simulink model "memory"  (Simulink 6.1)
settings: Solver=ode45  StartTime=0.0  StopTime=25.0  RelTol=1e-3
undefined symbols (not defined in the file or in its folder): Bit, Location, Lower, memory_netlist, Width
libraries: xbsIndex_r3 x19, adlibrary2 x2

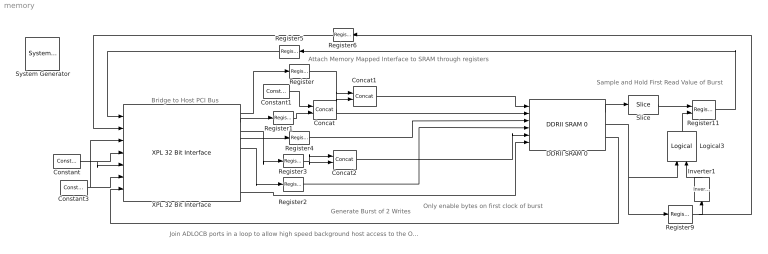
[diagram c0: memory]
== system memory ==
  note: Bridge to Host PCI Bus
  note: Attach Memory Mapped Interface to SRAM through registers
  note: Join ADLOCB ports in a loop to allow high speed background host access to the Off Chip Ram
  note: Generate Burst of 2 Writes
  note: Only enable bytes on first clock of burst
  note: Sample and Hold First Read Value of Burst
  " System Generator" : xbsIndex_r3/ System Generator  Tag=genX  xilinxfamily=Virtex2P  part=xc2vp70  speed=-6  package=ff1704  synthesis_tool=XST  directory=./memory_netlist  testbench=off  simulink_period=1  sysclk_period=10  incr_netlist=off  trim_vbits=Everywhere in SubSystem  dbl_ovrd=According to Block Masks  core_generation=According to Block Masks  run_coregen=off  deprecated_control=off  eval_field=0
  Concat : xbsIndex_r3/Concat  num_inputs=2  explicit_period=off  period=1  dbl_ovrd=off
  Concat1 : xbsIndex_r3/Concat  num_inputs=2  explicit_period=off  period=1  dbl_ovrd=off
  Concat2 : xbsIndex_r3/Concat  num_inputs=2  explicit_period=off  period=1  dbl_ovrd=off
  Constant : xbsIndex_r3/Constant  const=0  equ=P=C  arith_type=Boolean  n_bits=1  bin_pt=0  opselect=C  inp2=PCIN>>17  opr=+  inp1=P  carry=CIN  iostate=0  explicit_period=on  period=1  dbl_ovrd=off
  Constant1 : xbsIndex_r3/Constant  const=0  equ=P=C  arith_type=Unsigned  n_bits=5  bin_pt=0  opselect=C  inp2=PCIN>>17  opr=+  inp1=P  carry=CIN  iostate=0  explicit_period=on  period=1  dbl_ovrd=off
  Constant3 : xbsIndex_r3/Constant  const=0  equ=P=C  arith_type=Unsigned  n_bits=32  bin_pt=0  opselect=C  inp2=PCIN>>17  opr=+  inp1=P  carry=CIN  iostate=0  explicit_period=on  period=1  dbl_ovrd=off
  DDRII SRAM 0 : adlibrary2/ADM-XP/DDRII SRAM 0
  Inverter1 : xbsIndex_r3/Inverter  Orientation=up  latency=0  explicit_period=off  period=1  en=off  dbl_ovrd=off  show_param=off
  Logical3 : xbsIndex_r3/Logical  Orientation=up  logical_function=AND  inputs=2  precision=Full  arith_type=Unsigned  n_bits=8  bin_pt=2  align_bp=on  latency=0  explicit_period=off  period=1  en=off  dbl_ovrd=off  show_param=off
  Register{,1..4} (5 alike) : xbsIndex_r3/Register  init=0  reg_only_valid=off  explicit_period=on  period=1  rst=off  en=off  out_en=off  dbl_ovrd=off  show_param=off
  Register11 : xbsIndex_r3/Register  init=0  reg_only_valid=off  explicit_period=off  period=1  rst=off  en=on  out_en=off  dbl_ovrd=off  show_param=off
  Register5 : xbsIndex_r3/Register  Orientation=left  init=0  reg_only_valid=off  explicit_period=on  period=1  rst=off  en=off  out_en=off  dbl_ovrd=off  show_param=off
  Register6 : xbsIndex_r3/Register  Orientation=left  init=0  reg_only_valid=off  explicit_period=on  period=1  rst=off  en=off  out_en=off  dbl_ovrd=off  show_param=off
  Register9 : xbsIndex_r3/Register  init=0  reg_only_valid=off  explicit_period=off  period=1  rst=off  en=off  out_en=off  dbl_ovrd=off  show_param=off
  Slice : xbsIndex_r3/Slice  mode=Lower Bit Location + Width  nbits=32  bit1=0  base1=MSB of Input  bit0=0  base0=LSB of Input  boolean_output=off  explicit_period=off  period=1  dbl_ovrd=off
  XPL 32 Bit Interface : adlibrary2/ADM-XPL/XPL 32 Bit Interface  program='slave_write 0x0 0x1234;slave_read 0x0'  clock_ratio=1.5
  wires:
  Constant/1 -> XPL 32 Bit Interface/5, XPL 32 Bit Interface/4
  Constant3/1 -> XPL 32 Bit Interface/3, XPL 32 Bit Interface/6
  XPL 32 Bit Interface/5 -> Register2/1
  XPL 32 Bit Interface/2 -> Register1/1
  XPL 32 Bit Interface/1 -> Register/1
  Register/1 -> Concat1/2, Concat1/1
  Register4/1 -> DDRII SRAM 0/3
  Concat/1 -> DDRII SRAM 0/2
  Constant1/1 -> Concat/1
  Register1/1 -> Concat/2
  Register5/1 -> XPL 32 Bit Interface/1
  Register6/1 -> XPL 32 Bit Interface/2
  Concat1/1 -> DDRII SRAM 0/1
  Register3/1 -> Concat2/1, Concat2/2
  XPL 32 Bit Interface/4 -> Register4/1
  XPL 32 Bit Interface/3 -> Register3/1
  DDRII SRAM 0/3 -> XPL 32 Bit Interface/7
  XPL 32 Bit Interface/10 -> DDRII SRAM 0/6
  Register2/1 -> DDRII SRAM 0/4
  DDRII SRAM 0/1 -> Slice/1
  Slice/1 -> Register11/1
  Logical3/1 -> Register11/2
  Inverter1/1 -> Logical3/2
  DDRII SRAM 0/2 -> Register9/1, Logical3/1
  Register9/1 -> Inverter1/1, Register6/1
  Register11/1 -> Register5/1
  Concat2/1 -> DDRII SRAM 0/5
